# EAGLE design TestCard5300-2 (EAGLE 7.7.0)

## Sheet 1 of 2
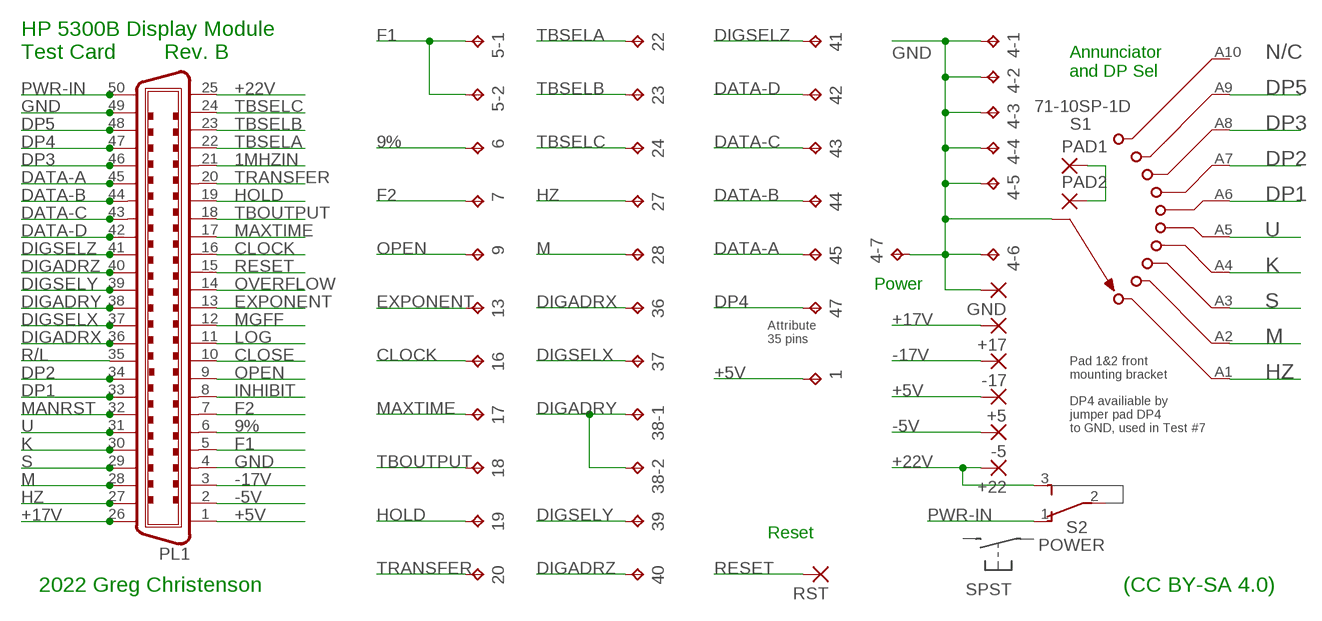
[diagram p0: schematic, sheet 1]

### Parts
1  TPPAD1-17  [P1-17]
4-1  TPPAD1-17  [P1-17]
4-2  TPPAD1-17  [P1-17]
4-3  TPPAD1-17  [P1-17]
4-4  TPPAD1-17  [P1-17]
4-5  TPPAD1-17  [P1-17]
4-6  TPPAD1-17  [P1-17]
4-7  TPPAD1-17  [P1-17]
5-1  TPPAD1-17  [P1-17]
5-2  TPPAD1-17  [P1-17]
6  TPPAD1-17  [P1-17]
7  TPPAD1-17  [P1-17]
9  TPPAD1-17  [P1-17]
13  TPPAD1-17  [P1-17]
16  TPPAD1-17  [P1-17]
17  TPPAD1-17  [P1-17]
18  TPPAD1-17  [P1-17]
19  TPPAD1-17  [P1-17]
20  TPPAD1-17  [P1-17]
22  TPPAD1-17  [P1-17]
23  TPPAD1-17  [P1-17]
24  TPPAD1-17  [P1-17]
27  TPPAD1-17  [P1-17]
28  TPPAD1-17  [P1-17]
36  TPPAD1-17  [P1-17]
37  TPPAD1-17  [P1-17]
38-1  TPPAD1-17  [P1-17]
38-2  TPPAD1-17  [P1-17]
39  TPPAD1-17  [P1-17]
40  TPPAD1-17  [P1-17]
41  TPPAD1-17  [P1-17]
42  TPPAD1-17  [P1-17]
43  TPPAD1-17  [P1-17]
44  TPPAD1-17  [P1-17]
45  TPPAD1-17  [P1-17]
47  TPPAD1-17  [P1-17]
+5  3,17/1,3  [3,17/1,3]
+17  3,17/1,3  [3,17/1,3]
+22  3,17/1,3  [3,17/1,3]
-5  3,17/1,3  [3,17/1,3]
-17  3,17/1,3  [3,17/1,3]
GND  3,17/1,3  [3,17/1,3]
PAD1  3,17/1,3  [3,17/1,3]
PAD2  3,17/1,3  [3,17/1,3]
PL1  C50H  [50H]
RST  3,17/1,3  [3,17/1,3]
S1  71-10SP-1D  [71-10-1D-1C]
S2  POWER  TL36PO  [TL3XPO]

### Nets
1MHZIN: PL1.21
9%: 6.TP PL1.6
+5V: 1.TP +5.1(P) PL1.1
+17V: +17.1(P) PL1.26
+22V: +22.1(P) PL1.25 S2.3(S)
-5V: -5.1(P) PL1.2
-17V: -17.1(P) PL1.3
CLOCK: 16.TP PL1.16
CLOSE: PL1.10
DATA-A: 45.TP PL1.45
DATA-B: 44.TP PL1.44
DATA-C: 43.TP PL1.43
DATA-D: 42.TP PL1.42
DIGADRX: 36.TP PL1.36
DIGADRY: 38-1.TP 38-2.TP PL1.38
DIGADRZ: 40.TP PL1.40
DIGSELX: 37.TP PL1.37
DIGSELY: 39.TP PL1.39
DIGSELZ: 41.TP PL1.41
DP1: PL1.33 S1.A6
DP2: PL1.34 S1.A7
DP3: PL1.46 S1.A8
DP4: 47.TP PL1.47
DP5: PL1.48 S1.A9
EXPONENT: 13.TP PL1.13
F1: 5-1.TP 5-2.TP PL1.5
F2: 7.TP PL1.7
GND: 4-1.TP 4-2.TP 4-3.TP 4-4.TP 4-5.TP 4-6.TP 4-7.TP GND.1(P) PAD1.1(P) PAD2.1(P) PL1.4 PL1.49 S1.A-COM(COM)
HOLD: 19.TP PL1.19
HZ: 27.TP PL1.27 S1.A1
INHIBIT: PL1.8
K: PL1.30 S1.A4
LOG: PL1.11
M: 28.TP PL1.28 S1.A2
MANRST: PL1.32
MAXTIME: 17.TP PL1.17
MGFF: PL1.12
OPEN: 9.TP PL1.9
OVERFLOW: PL1.14
PWR-IN: PL1.50 S2.1(O)
R/L: PL1.35
RESET: PL1.15 RST.1(P)
S: PL1.29 S1.A3
TBOUTPUT: 18.TP PL1.18
TBSELA: 22.TP PL1.22
TBSELB: 23.TP PL1.23
TBSELC: 24.TP PL1.24
TRANSFER: 20.TP PL1.20
U: PL1.31 S1.A5
Unconnected: S1.A10 S2.2(P)

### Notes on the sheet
- HP 5300B Display Module
  Test Card        Rev. B
- N/C
- Annunciator
  and DP Sel
- Power
- Attribute
  35 pins
- Pad 1&2 front
  mounting bracket
- DP4 availiable by
  jumper pad DP4
  to GND, used in Test #7
- Reset
- 2022 Greg Christenson | (CC BY-SA 4.0)

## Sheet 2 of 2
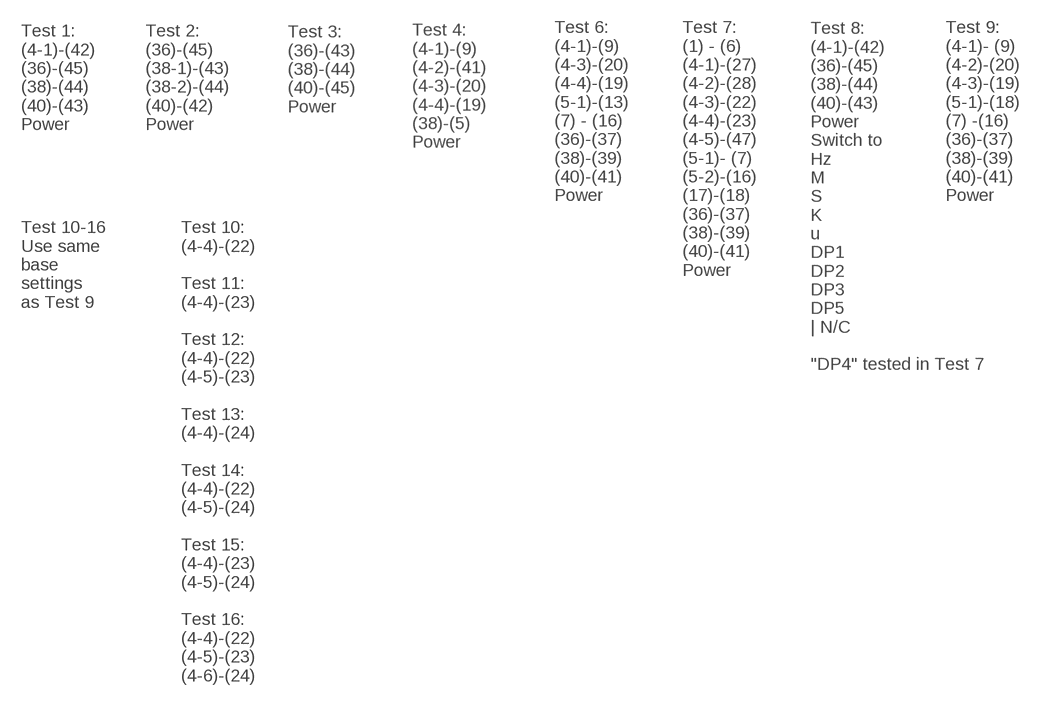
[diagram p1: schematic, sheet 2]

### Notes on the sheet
- Test 3:
  (36)-(43)
  (38)-(44)
  (40)-(45)
  Power
- Test 1:
  (4-1)-(42)
  (36)-(45)
  (38)-(44)
  (40)-(43)
  Power
- Test 2:
  (36)-(45)
  (38-1)-(43)
  (38-2)-(44)
  (40)-(42)
  Power
- Test 4:
  (4-1)-(9)
  (4-2)-(41)
  (4-3)-(20)
  (4-4)-(19)
  (38)-(5)
  Power
- Test 6:
  (4-1)-(9)
  (4-3)-(20)
  (4-4)-(19)
  (5-1)-(13)
  (7) - (16)
  (36)-(37)
  (38)-(39)
  (40)-(41)
  Power
- Test 9:
  (4-1)- (9)
  (4-2)-(20)
  (4-3)-(19)
  (5-1)-(18)
  (7) -(16)
  (36)-(37)
  (38)-(39)
  (40)-(41)
  Power
- Test 7:
  (1) - (6)
  (4-1)-(27)
  (4-2)-(28)
  (4-3)-(22)
  (4-4)-(23)
  (4-5)-(47)
  (5-1)- (7)
  (5-2)-(16)
  (17)-(18)
  (36)-(37)
  (38)-(39)
  (40)-(41)
  Power
- Test 10-16
  Use same
  base
  settings
  as Test 9
- Test 8:
  (4-1)-(42)
  (36)-(45)
  (38)-(44)
  (40)-(43)
  Power
  Switch to
  Hz
  M
  S
  K
  u
  DP1
  DP2
  DP3
  DP5
  | N/C
  
  "DP4" tested in Test 7
- Test 10:
  (4-4)-(22)
  
  Test 11:
  (4-4)-(23)
  
  Test 12:
  (4-4)-(22)
  (4-5)-(23)
  
  Test 13:
  (4-4)-(24)
  
  Test 14:
  (4-4)-(22)
  (4-5)-(24)
  
  Test 15:
  (4-4)-(23)
  (4-5)-(24)
  
  Test 16:
  (4-4)-(22)
  (4-5)-(23)
  (4-6)-(24)

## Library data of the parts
1 47 = testpad:TP: Test pad; DESC: Pin Receptacle Connector 0.020" ~ 0.032" Mtg-hole=1.45mm; MFG: Mill-Max; PN: 0338-0-15-15-15-27-10-0
4-1-4-7 5-1 5-2 6 7 9 13 16-20 22-24 27 28 36 37 38-1 38-2 39-45 = testpad:TP: Test pad
+5 +17 +22 -5 -17 GND RST = wirepad:3,17/1,3: THROUGH-HOLE PAD; DESC: TERM TURRET SINGLE L=5.84mm Mt-Hole=1.3mm TIN; MFG: Mill-Max; PN: 2110-2-00-80-00-00-07-0
PAD1 PAD2 = wirepad:3,17/1,3: THROUGH-HOLE PAD
PL1 = con-amp-champ:C50H: CONNECTOR; DESC: CONN SCSI RCPT 50POS R/A SOLDER; MFG: NorComp Inc.; OC_FARNELL: unknown; OC_NEWARK: unknown; PN: 112-050-213R001
S1 = switch-grayhill:71-10SP-1D: Rotary Switch Grayhill 71 Series, 10 Pos, 1 Pole, 1 Deck; DESC: SWITCH ROTARY 2-10POS 250MA 115V; MFG: Grayhill; PN: 71BDF36-01-1-AJN
S2 = switch:TL36PO: TINY SWITCH ON - ON Source: http://www2.produktinfo.conrad.com/datenblaetter/700000-724999/705152-da-01-de-Subminiaturschalter_TL_36YO.pdf; DESC: SWITCH TOGGLE SPST 0.4VA 28V Through Hole; MFG: NKK Switches; PN: A11JP

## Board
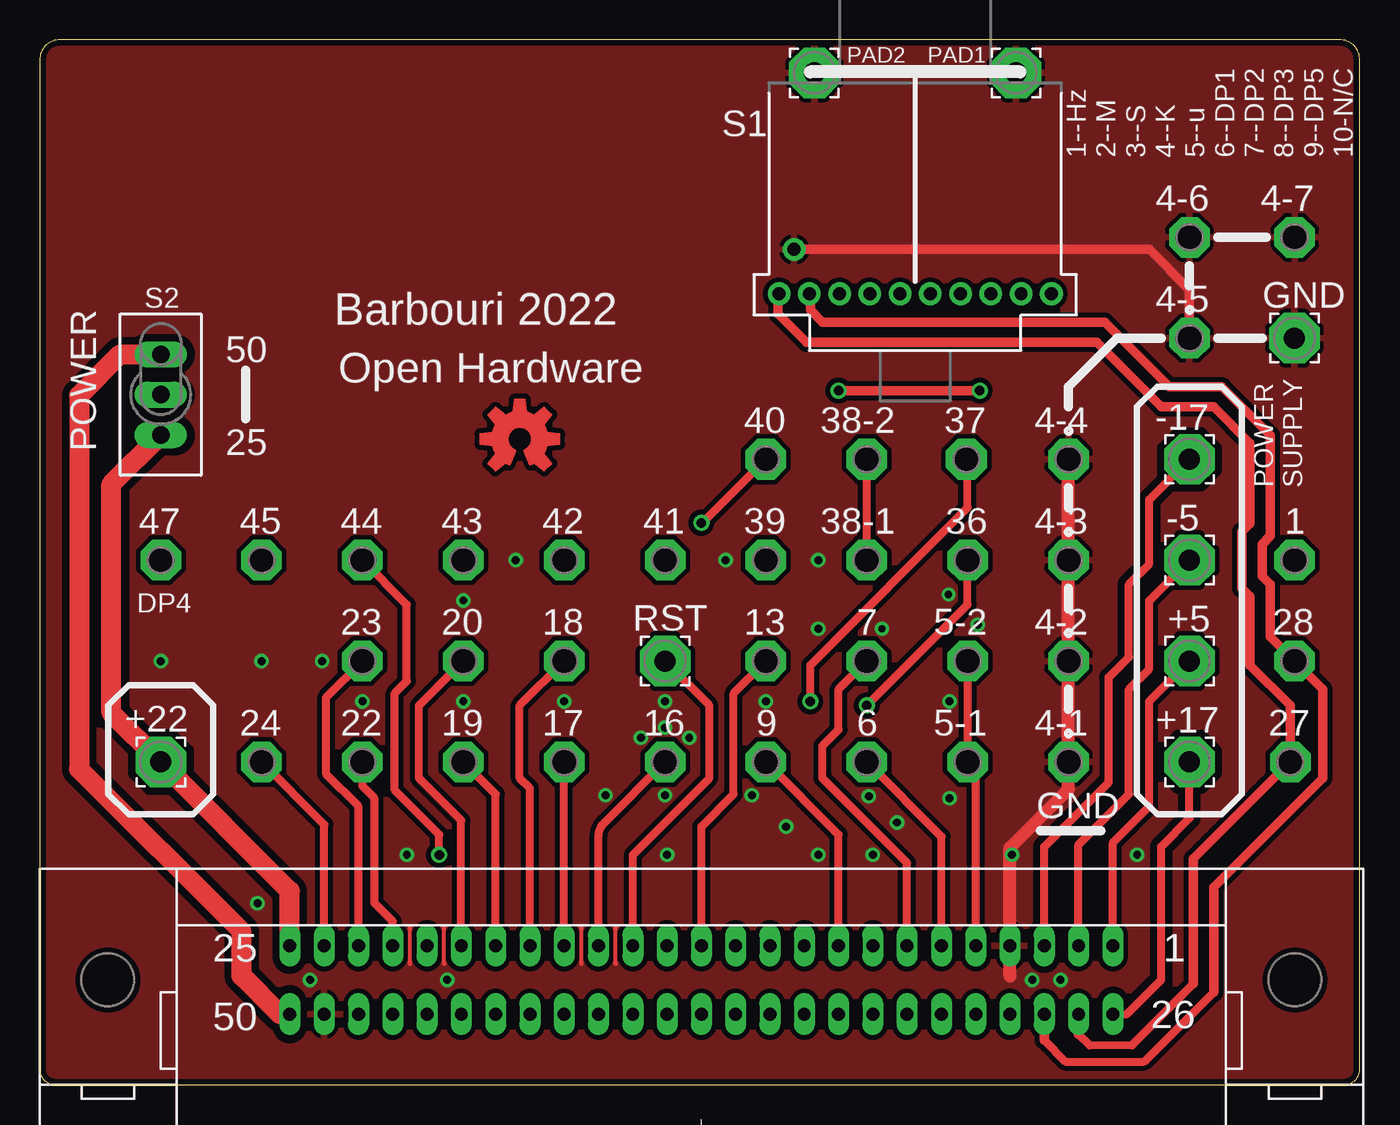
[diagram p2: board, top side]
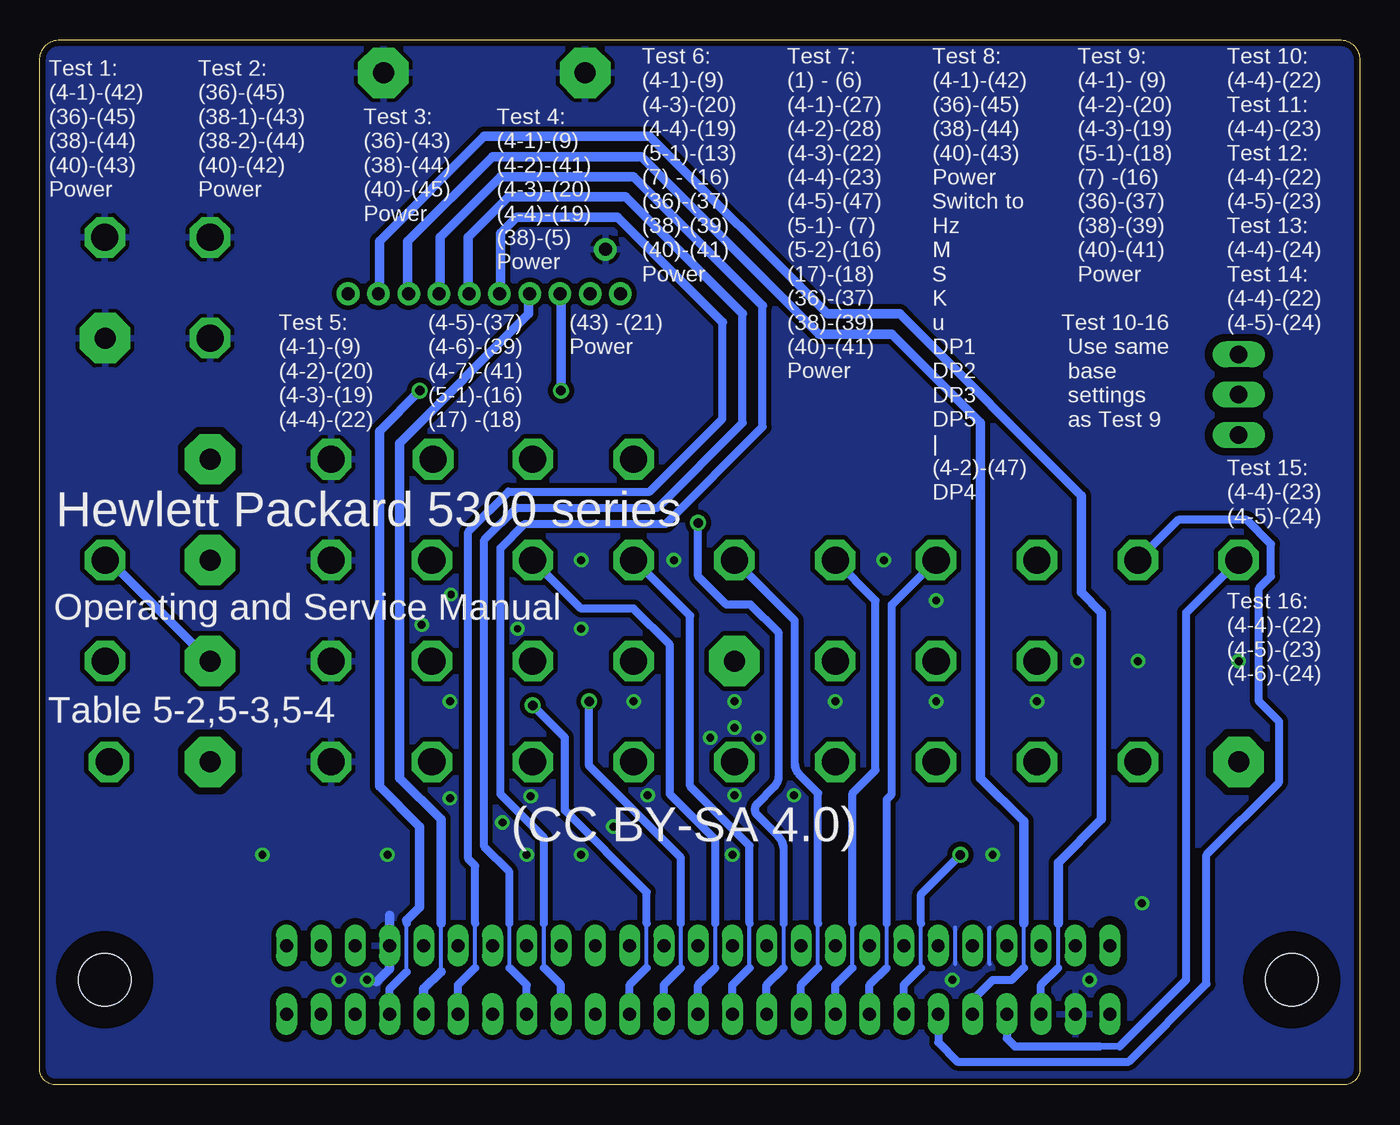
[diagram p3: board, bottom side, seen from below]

Size 83.11 x 65.77 mm. Coordinates in mm from the lower left corner, seen from the top.
Outline: 0,64.5 0,1 arc90 1,0 82.11,0 arc90 83.11,1 83.11,64.5 arc90 81.84,65.77 1.27,65.77 arc90 0,64.5
Copper layers (1*16): Top 0.035mm / dielectric 1.5mm / Bottom 0.035mm
Design rules "default *": minimum track width 12mil, minimum drill 9mil, track to track 12mil, track to pad 12mil, pad to pad 12mil, via to via 12mil, smd to smd 8mil, copper to edge 15mil, drill to drill 9mil, minimum pad ring 10mil, minimum via ring 8mil, stop-mask expansion 4mil, vias tented up to drill 24mil, thermal gap 10mil
tRestrict: 53 lines
bRestrict: 31 lines

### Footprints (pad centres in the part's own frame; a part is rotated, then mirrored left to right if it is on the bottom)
P1-17 = drill 1.702 pad 2.54 octagon: TP 0,0
3,17/1,3 = drill 1.321 pad 3.175 octagon: 1 0,0
50H = drill 0.813 long: 1 -25.908,-2.159; 2 -23.749,-2.159; 3 -21.59,-2.159; 4 -19.431,-2.159; 5 -17.272,-2.159; 6 -15.113,-2.159; 7 -12.954,-2.159; 8 -10.795,-2.159; 9 -8.636,-2.159; 10 -6.477,-2.159; 11 -4.318,-2.159; 12 -2.159,-2.159; 13 0,-2.159; 14 2.159,-2.159; 15 4.318,-2.159; 16 6.477,-2.159; 17 8.636,-2.159; 18 10.795,-2.159; 19 12.954,-2.159; 20 15.113,-2.159; 21 17.272,-2.159; 22 19.431,-2.159; 23 21.59,-2.159; 24 23.749,-2.159; 25 25.908,-2.159; 26 -25.908,2.159; 27 -23.749,2.159; 28 -21.59,2.159; 29 -19.431,2.159; 30 -17.272,2.159; 31 -15.113,2.159; 32 -12.954,2.159; 33 -10.795,2.159; 34 -8.636,2.159; 35 -6.477,2.159; 36 -4.318,2.159; 37 -2.159,2.159; 38 0,2.159; 39 2.159,2.159; 40 4.318,2.159; 41 6.477,2.159; 42 8.636,2.159; 43 10.795,2.159; 44 12.954,2.159; 45 15.113,2.159; 46 17.272,2.159; 47 19.431,2.159; 48 21.59,2.159; 49 23.749,2.159; 50 25.908,2.159 | hole 3.302: -37.363,0; 37.363,0
71-10-1D-1C = drill 0.813 pad 1.422: A1 2.794,-8.572; A2 2.794,-6.668; A3 2.794,-4.763; A4 2.794,-2.857; A5 2.794,-0.953; A6 2.794,0.953; A7 2.794,2.857; A8 2.794,4.763; A9 2.794,6.668; A10 2.794,8.572; A-COM 0,-7.62
TL3XPO = drill 1.1 pad 1.422 long: 1 -2.54,0; 2 0,0; 3 2.54,0

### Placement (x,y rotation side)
1  78.99,33.02 0 top
4-1  64.77,20.32 0 top
4-2  64.77,26.67 0 top
4-3  64.77,33.02 0 top
4-4  64.77,39.37 0 top
4-5  72.39,46.99 0 top
4-6  72.39,53.34 0 top
4-7  79.01,53.34 0 top
5-1  58.42,20.32 0 top
5-2  58.42,26.67 0 top
6  52.07,20.32 0 top
7  52.07,26.67 0 top
9  45.72,20.32 0 top
13  45.72,26.67 0 top
16  39.37,20.32 0 top
17  33.02,20.32 0 top
18  33.02,26.67 0 top
19  26.67,20.32 0 top
20  26.67,26.67 0 top
22  20.32,20.32 0 top
23  20.32,26.67 0 top
24  13.97,20.32 0 top
27  78.74,20.32 0 top
28  78.99,26.67 0 top
36  58.42,33.02 0 top
37  58.34,39.37 0 top
38-1  52.07,33.02 0 top
38-2  52.07,39.37 0 top
39  45.72,33.02 0 top
40  45.72,39.37 0 top
41  39.37,33.02 0 top
42  33.02,33.02 0 top
43  26.67,33.02 0 top
44  20.32,33.02 0 top
45  13.97,33.02 0 top
47  7.62,33.02 0 top
+5  72.39,26.67 0 top
+17  72.39,20.32 0 top
+22  7.62,20.32 0 top
-5  72.39,33.02 0 top
-17  72.39,39.37 0 top
GND  78.99,46.99 0 top
PAD1  61.47,63.69 0 top
PAD2  48.77,63.69 0 top
PL1  41.66,6.6 180 top
RST  39.37,26.67 0 top
S1  55.12,52.58 270 top
S2  7.62,43.43 270 top
U$2  [OSHW-LOGO-M_COPPER]  30.23,40.64 0 top

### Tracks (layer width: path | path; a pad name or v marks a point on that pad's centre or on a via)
9%
  Top 0.508: PL1.6 56.77,15.62 6.TP
+5V
  Top 0.508: PL1.1 67.56,15.24 69.85,17.53 69.85,24.13 +5.1
  Bottom 0.508: 78.49,32.77 78.74,32.77 1.TP
  Bottom 0.61: +5.1 78.49,32.77
+17V
  Top 0.508: PL1.26 68.45,4.45 70.61,6.6 70.61,14.99 72.39,16.76 +17.1
+22V
  Top 1.27: PL1.25 15.75,12.19 +22.1 4.51,23.43 4.51,37.78 S2.3
-5V
  Top 0.508: PL1.2 65.41,15.11 68.58,18.29 68.58,24.89 69.85,26.16 69.85,30.48 -5.1
-17V
  Top 0.508: PL1.3 63.25,14.99 67.31,19.05 67.31,25.65 68.58,26.92 68.58,31.5 69.85,32.77 69.85,36.83 -17.1
CLOCK
  Top 0.508: PL1.16 35.18,15.6 arc-45 35.55,16.5 16.TP
DATA-A
  Bottom 0.508: PL1.45 26.54,2.67 25.34,1.46 14.54,1.46 9.65,6.35 9.65,14.48 5.08,19.05 5.08,22.86 6.35,24.13 6.35,31.24 5.59,32 5.59,34.04 7.11,35.56 11.43,35.56 45.TP
DATA-B  (via drill 0.6)
  Top 0.508: v25.15,14.48 25.15,15.75 22.35,18.54 22.35,24.64 23.11,25.4 23.11,30.23 44.TP
  Bottom 0.254: 27.62,7.37 27.62,10.16
  Bottom 0.508: PL1.44 28.7,6.29 27.62,7.37 | 27.62,10.16 27.62,12 v25.15,14.48
DATA-C
  Bottom 0.254: 29.78,7.37 29.78,10.16
  Bottom 0.508: PL1.43 30.86,6.29 29.78,7.37 | 29.78,10.16 29.78,17.97 29.46,18.29 29.46,30.23 43.TP
DATA-D
  Bottom 0.254: 31.94,7.37 31.94,10.16
  Bottom 0.508: PL1.42 33.02,6.29 31.94,7.37 | 31.94,10.16 31.94,18.35 30.48,19.81 30.48,30.48 42.TP
DIGADRX  (via drill 0.6)
  Top 0.508: v52.07,23.88 58.42,30.23 36.TP
  Bottom 0.254: 44.9,7.37 44.9,10.16
  Bottom 0.508: PL1.36 45.97,6.29 44.9,7.37 | 44.9,10.16 44.9,12.13 50.04,17.27 50.04,21.84 v52.07,23.88
DIGADRY
  Top 0.508: 38-1.TP 38-2.TP
  Bottom 0.254: 40.58,7.37 40.58,10.16
  Bottom 0.508: PL1.38 41.66,6.29 40.58,7.37 | 40.58,10.16 40.58,15.43 43.43,18.29 43.43,27.69 45.72,29.97 49.02,29.97 38-1.TP
DIGADRZ  (via drill 0.6)
  Top 0.508: v41.66,35.37 41.97,35.62 40.TP
  Bottom 0.254: 36.26,7.37 36.26,10.16
  Bottom 0.508: PL1.40 37.34,6.29 36.26,7.37 | 36.26,10.16 36.26,14.78 arc-45 36.63,15.68 37.93,16.98 arc90 37.93,17.7 36.87,18.76 arc-45 36.58,19.46 36.58,28.45 38.35,30.23 39.88,30.23 41.66,32 v41.66,35.37
DIGSELX  (via drill 0.6)
  Top 0.508: v48.51,24.13 48.51,26.42 58.42,36.32 58.42,39.29 37.TP
  Bottom 0.254: 42.74,7.37 42.74,10.16
  Bottom 0.508: PL1.37 43.81,6.29 42.74,7.37 | 42.74,10.16 42.74,14.29 48.51,20.07 v48.51,24.13
DIGSELY
  Bottom 0.254: 38.42,7.37 38.42,10.16
  Bottom 0.508: PL1.39 39.5,6.29 38.42,7.37 | 38.42,10.16 38.42,15.05 42.16,18.8 42.16,29.53 45.66,33.02 39.TP
DIGSELZ
  Bottom 0.254: 34.1,7.37 34.1,10.16
  Bottom 0.508: PL1.41 35.18,6.29 34.1,7.37 | 34.1,10.16 34.1,18.35 35.27,19.52 arc45 35.56,20.23 35.56,29.21 41.TP
DP1
  Bottom 0.254: 53.53,7.37 53.53,10.16
  Bottom 0.508: PL1.33 52.45,6.29 53.53,7.37 | 53.53,10.16 53.53,13.4 55.12,14.99 55.12,34.29 53.09,36.32 44.2,36.32 38.86,41.66 38.86,48.51 | 56.13,49.85 S1.A6
  Bottom 0.61: 38.86,48.51 46.23,55.88 53.59,55.88 56.13,53.34 56.13,49.85
DP2
  Bottom 0.254: 51.37,7.37 51.37,10.16
  Bottom 0.508: PL1.34 50.29,6.29 51.37,7.37 | 51.37,10.16 51.37,15.56 54.1,18.29 54.1,33.78 52.58,35.31 43.69,35.31 37.59,41.4 37.59,49.02 | 57.91,49.85 S1.A7
  Bottom 0.61: 37.59,49.02 45.72,57.15 54.1,57.15 57.91,53.34 57.91,49.85
DP3
  Bottom 0.254: 21.14,7.37 21.14,10.16
  Bottom 0.508: PL1.46 24.38,5.33 23.11,6.6 21.91,6.6 21.14,7.37 | 59.94,49.85 S1.A8
  Bottom 0.61: 59.94,49.85 59.94,53.09 54.61,58.42 45.21,58.42 34.04,47.24 29.46,47.24 23.88,41.66 23.88,19.3 21.14,16.57 21.14,10.16
DP4
  Bottom 0.406: 16.38,2.41 15.11,2.41
  Bottom 0.508: PL1.47 22.23,2.92 21.72,2.41 16.38,2.41 | 15.11,2.41 10.92,6.6 10.92,29.72 47.TP
DP5
  Bottom 0.254: 18.99,7.37 18.99,10.16
  Bottom 0.508: PL1.48 20.07,6.29 18.99,7.37 | 61.72,49.85 S1.A9
  Bottom 0.61: 18.99,10.16 18.99,13.97 16.26,16.7 16.26,29.72 17.53,30.99 17.53,37.08 28.96,48.51 33.53,48.51 44.7,59.69 55.12,59.69 61.72,53.09 61.72,49.85
EXPONENT
  Top 0.508: PL1.13 41.66,16.26 43.69,18.29 43.69,24.64 13.TP
F1
  Top 0.508: PL1.5 58.93,19.81 5-1.TP 5-2.TP
F2
  Top 0.508: PL1.7 54.61,13.97 49.28,19.3 49.28,21.34 50.29,22.35 50.29,24.89 7.TP
GND  (via drill 0.45, 0.5)
  Top 0.254: 25.46,7.62 25.46,9.97 | 23.3,7.62 23.3,9.97 | 34.1,7.62 34.1,9.91 | 36.26,7.62 36.26,9.91
  Top 0.61: 4-5.TP 72.39,50.04 69.85,52.58 S1.A-COM
  Top 0.813: 4-4.TP 4-3.TP 4-2.TP 4-1.TP 64.77,18.61 61.09,14.92 61.09,6.86
  Bottom 0.254: 25.46,7.62 25.46,9.91 | 23.3,7.62 23.3,9.91
  Bottom 0.61: 61.09,10.67 61.09,7.3 61.91,6.48
  other vias: 7.62,26.67 13.97,26.67 17.78,26.67 29.97,33.02 26.67,24.13 33.02,24.13 39.37,24.13 26.67,30.48 49.02,33.02 43.18,33.02 49.02,28.7 45.72,24.13 46.99,16.26 49.02,14.48 23.11,14.48 25.65,6.6 57.28,24.13 57.28,18.03 62.48,6.6 64.26,6.6 53.02,28.7 57.21,30.86 52.45,14.48 53.98,16.51 52.2,18.16 61.21,14.48 13.72,11.43 17.02,6.6 69.09,14.48 59.05,28.96 20.32,24.13 39.5,14.48 44.83,18.22 35.62,18.22 39.37,18.22 37.85,21.84 40.89,21.84 39.37,22.48
  pour Top: 0,0 83.11,0 83.11,65.79 0,65.79
  pour Bottom: 0,0 83.11,0 83.11,65.79 0,65.79
HOLD
  Top 0.508: PL1.19 28.7,18.29 19.TP
HZ
  Top 0.457: 66.1,2.48 68.77,2.48
  Top 0.508: 65.41,3.17 66.1,2.48 | 68.77,2.48 72.64,6.35 | 46.48,49.72 S1.A1
  Top 0.61: PL1.27 65.41,3.17 | 72.64,6.35 72.64,14.22 27.TP 78.74,23.88 76.2,26.42 76.2,30.73 75.69,31.24 75.69,34.8 76.2,35.31 76.2,40.39 73.91,42.67 70.61,42.67 66.55,46.74 48.26,46.74 46.48,48.51 46.48,49.72
K
  Bottom 0.254: 57.85,7.11 57.85,10.16
  Bottom 0.508: 52.32,49.72 S1.A4
  Bottom 0.61: PL1.30 58.93,6.03 57.85,7.11 | 57.85,10.16 57.85,16.7 60.45,19.3 60.45,40.39 52.32,48.51 52.32,49.72
M
  Top 0.508: 63.25,2.79 64.58,1.46 69.53,1.46 73.91,5.84 | 48.51,49.72 S1.A2
  Top 0.61: PL1.28 63.25,2.79 | 73.91,5.84 73.91,12.45 80.77,19.3 80.77,24.89 28.TP 77.47,28.19 77.47,31.5 76.96,32 76.96,34.04 77.47,34.54 77.47,40.89 74.42,43.94 71.12,43.94 67.06,48.01 49.28,48.01 48.51,48.77 48.51,49.72
MAXTIME
  Top 0.508: PL1.17 17.TP
OPEN
  Top 0.508: PL1.9 50.29,15.75 9.TP
PWR-IN
  Top 1.27: PL1.50 15.11,4.45 12.7,6.86 12.7,9.65 2.48,19.88 2.48,43.37 5.08,45.97 S2.1
RESET
  Top 0.508: PL1.15 37.34,14.48 42.16,19.3 42.16,23.88 RST.1
S  (via drill 0.6)
  Top 0.61: v59.18,43.69 v50.29,43.69
  Bottom 0.254: 60.01,7.11 60.01,10.16
  Bottom 0.508: PL1.29 61.09,6.03 60.01,7.11 | 60.01,10.16 60.01,10.35 | 50.29,49.72 S1.A3
  Bottom 0.61: 60.01,10.35 59.18,11.18 59.18,16.26 61.72,18.8 61.72,41.15 v59.18,43.69 | v50.29,43.69 50.29,49.72
TBOUTPUT
  Top 0.508: PL1.18 30.86,18.67 30.23,19.3 30.23,23.88 18.TP
TBSELA
  Top 0.508: PL1.22 22.23,10.29 21.08,11.43 21.08,18.03 20.32,18.8 22.TP
TBSELB
  Top 0.508: PL1.23 20.07,17.53 18.03,19.56 18.03,24.38 23.TP
TBSELC
  Top 0.508: PL1.24 17.91,16.38 24.TP
TRANSFER
  Top 0.508: PL1.20 26.54,16.64 23.88,19.3 23.88,23.88 20.TP
U
  Bottom 0.254: 55.69,7.37 55.69,10.16
  Bottom 0.508: PL1.31 56.77,6.29 55.69,7.37 | 55.69,10.16 55.69,13.78 56.13,14.22 56.13,34.8 53.59,37.34 44.7,37.34 40.13,41.91 40.13,48.01 | 54.1,49.85 S1.A5
  Bottom 0.61: 40.13,48.01 46.74,54.61 53.09,54.61 54.1,53.59 54.1,49.85

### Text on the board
tNames: 1--Hz / 2--M / 3--S / 4--K / 5--u / 6--DP1 / 7--DP2 / 8--DP3 / 9--DP5 / 10-N/C | Barbouri 2022 | 50 | Open Hardware | 25 | POWER / SUPPLY | DP4 | GND
bNames: Test 2: / (36)-(45) / (38-1)-(43) / (38-2)-(44) / (40)-(42) / Power | Test 1: / (4-1)-(42) / (36)-(45) / (38)-(44) / (40)-(43) / Power | Test 3: / (36)-(43) / (38)-(44) / (40)-(45) / Power | Test 9: / (4-1)- (9) / (4-2)-(20) / (4-3)-(19) / (5-1)-(18) / (7) -(16) / (36)-(37) / (38)-(39) / (40)-(41) / Power | Test 6: / (4-1)-(9) / (4-3)-(20) / (4-4)-(19) / (5-1)-(13) / (7) - (16) / (36)-(37) / (38)-(39) / (40)-(41) / Power | Test 4: / (4-1)-(9) / (4-2)-(41) / (4-3)-(20) / (4-4)-(19) / (38)-(5) / Power | Test 10: / (4-4)-(22) / Test 11: / (4-4)-(23) / Test 12: / (4-4)-(22) / (4-5)-(23) / Test 13: / (4-4)-(24) / Test 14: / (4-4)-(22) / (4-5)-(24) | (43) -(21) / Power | Test 7: / (1) - (6) / (4-1)-(27) / (4-2)-(28) / (4-3)-(22) / (4-4)-(23) / (4-5)-(47) / (5-1)- (7) / (5-2)-(16) / (17)-(18) / (36)-(37) / (38)-(39) / (40)-(41) / Power | Test 10-16 / Use same / base / settings / as Test 9 | (4-5)-(37) / (4-6)-(39) / (4-7)-(41) / (5-1)-(16) / (17) -(18) | Test 5: / (4-1)-(9) / (4-2)-(20) / (4-3)-(19) / (4-4)-(22) | Test 8: / (4-1)-(42) / (36)-(45) / (38)-(44) / (40)-(43) / Power / Switch to / Hz / M / S / K / u / DP1 / DP2 / DP3 / DP5 / | / (4-2)-(47) / DP4 | Test 15: / (4-4)-(23) / (4-5)-(24) | Hewlett Packard 5300 series | Operating and Service Manual | Test 16: / (4-4)-(22) / (4-5)-(23) / (4-6)-(24) | Table 5-2,5-3,5-4 | (CC BY-SA 4.0)
tStop: HP 5300 A/B / Display Module / Test Card / Rev. B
